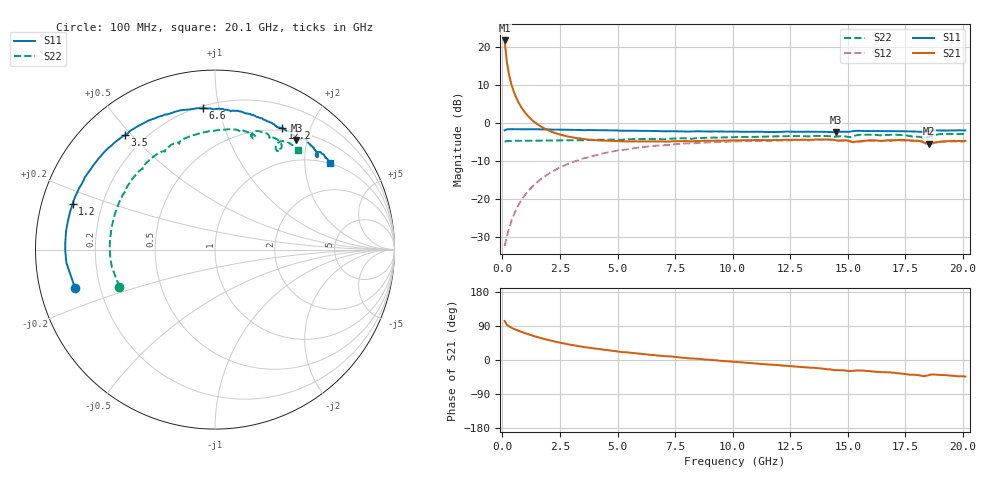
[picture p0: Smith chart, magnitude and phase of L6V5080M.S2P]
!  Infineon Technologies AG
! BFR380L3 , PF131585-7, No.6, Th 09.10.01, soldered on pcb-board, measured with PP GSG850
!  Vce=0.5 V,  Ic=80.0 mA
! Common Emitter S-Parameters:  15. November 2001
#  GHz  S  MA  R  50
! f  S11  S21  S12  S22
! GHz  Mag  Ang  Mag  Ang  Mag  Ang  Mag  Ang
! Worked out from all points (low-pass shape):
!   201 points, 100 MHz to 20.1 GHz, reference 50 ohm
!   highest |S21| = 21.83 dB at 100 MHz (marker M1); lowest = -5.4 dB at 18.5 GHz (marker M2)
!   |S21| within 3 dB of the highest: start of sweep to 151.8 MHz
!   lowest |S11| = -2.4 dB at 14.5 GHz (marker M3), VSWR 7.36, Z = 31.3 + j90.9 ohm
!   |S11| at or under -10 dB: nowhere
!   |S22| runs from -4.9 to -2.8 dB; largest |S21 - S12| = 12
!   S11 on the Smith chart (normalised r, x): 100 MHz: 0.11, -0.13; 1.2 GHz: 0.09, +0.16; 3.5 GHz: 0.13, +0.48; 6.6 GHz: 0.21, +0.90; 12.2 GHz: 0.47, +1.59; 20.1 GHz: 0.97, +2.67
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0.1  0.8086 -164.6  12.35 103.0  0.02393 41.8  0.572 -158.7
0.2  0.8312 -174.9  6.342 93.1  0.03204 51.2  0.5829 -170.6
0.3  0.834 -179.2  4.273 88.6  0.04172 57.9  0.5849 -175.4
0.4  0.8349 177.8  3.225 85.2  0.05198 61.8  0.5858 -178.3
0.5  0.8346 175.3  2.601 82.2  0.06213 64.5  0.5865 179.6
0.6  0.8362 173.1  2.182 79.7  0.07289 65.8  0.5869 177.9
0.7  0.835 171.1  1.891 77.2  0.08331 66.5  0.5871 176.3
0.9  0.834 167.5  1.5 72.6  0.1044 66.9  0.5877 173.6
1.2  0.8334 162.2  1.172 66.5  0.1356 65.9  0.5884 170.0
1.6  0.8312 155.7  0.9372 59.1  0.1762 63.3  0.5894 165.6
2.1  0.8262 147.9  0.7812 51.2  0.2244 59.1  0.592 160.4
3.5  0.811 128.1  0.6226 34.7  0.3429 46.1  0.5945 146.6
6.6  0.7907 94.7  0.5757 12.9  0.5022 20.2  0.6218 119.6
6.8  0.7869 92.9  0.5754 11.6  0.509 18.6  0.6195 117.9
10.1  0.7755 70.8  0.5931 -5.0  0.5742 -1.9  0.6549 96.3
12.2  0.773 61.2  0.6038 -14.9  0.5932 -12.8  0.674 84.0
13.5  0.7736 55.7  0.6088 -20.5  0.598 -19.3  0.6763 77.1
14.5  0.7609 53.4  0.5936 -26.8  0.5877 -25.8  0.6659 72.5
16.8  0.7859 45.4  0.5978 -32.4  0.587 -32.0  0.7035 62.5
18.2  0.7669 42.2  0.5776 -41.9  0.57 -41.4  0.6533 56.9
18.5  0.7906 43.6  0.5375 -40.4  0.5282 -39.3  0.6662 59.4
20.1  0.8047 37.1  0.5861 -43.8  0.5777 -43.3  0.7228 50.3
